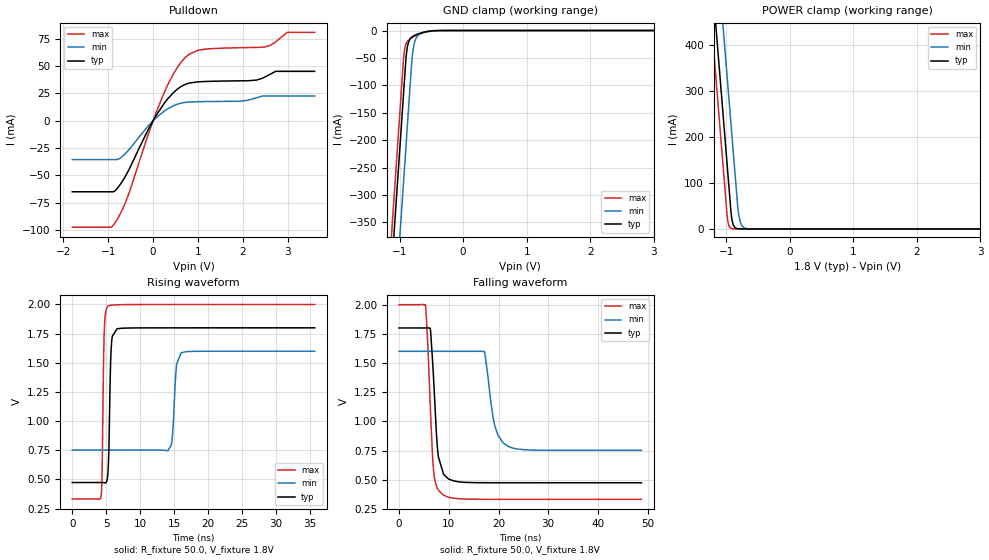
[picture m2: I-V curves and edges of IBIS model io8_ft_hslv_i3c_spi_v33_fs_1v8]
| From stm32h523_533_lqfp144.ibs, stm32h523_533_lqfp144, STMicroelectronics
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[Model]   io8_ft_hslv_i3c_spi_v33_fs_1v8
Model_type I/O_open_drain
Polarity   Non-Inverting
Enable   Active-Low
| CAP_THRESHOLD on pad IOFT is "UDTCAPC" :
| Rising=20.0% of vddiom   Falling=80.0% of vddiom
| C_comp min and max val. don't necessarily correlate with the min and max pvt
| but are the smallest and greatest pad capacitance found.
| var   typ   min   max
C_comp   3.69213pF  3.66975pF  3.86731pF
|C_comp_pulldown   3.69213pF  3.66975pF  3.86731pF
Vinl = 800.0mV
Vinh = 1.0V
Vmeas = 900.0mV   | Reference voltage for timing measurements
Cref  = 50.0pF   | Timing specification test load capacitance value
Rref  = 1.0MOhm   | Timing specification test load resistance value
Vref  = 990.0mV   | Timing specification test load voltage
[Model Spec]
| TIME_THRESHOLD on pin ZII2CV11 is "CMOS" :
| Rising=40.0% of vdd   Falling=60.0% of vdd
Vinl 693.80000mV 621.80000mV 774.80000mV
Vinh 1.05820V 933.20000mV 1.16320V
| variable   typ   min   max
[Temperature Range] 25.0 125.0 -40.0
| variable   typ   min   max
[Voltage Range] 1.8V 1.6V 2.0V
| variable   typ   min   max
[POWER Clamp Reference] 1.8V 1.6V 2.0V
| variable   typ   min   max
[GND Clamp Reference] 0V 0V 0V
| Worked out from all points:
|   slope of the pulldown table from 0 to 0.27 V, typ, clamps not added: 15.8 ohm
|   GND clamp passes 1 mA (typ) near -0.52 V on its own axis
|   POWER clamp passes 1 mA (typ) near -0.84 V on its own axis
|   rising waveform, R_fixture 50.0, V_fixture 1.8V: 20-80 % time 287ps typ, 468ps min, 243ps max; typ from 0.474 V to 1.8 V
|   falling waveform, R_fixture 50.0, V_fixture 1.8V: 20-80 % time 1.08ns typ, 1.84ns min, 1.02ns max; typ from 1.8 V to 0.474 V
[POWER Clamp]
-1.8V     1.518A     1.709A     1.407A
-1.23V    548.8mA    740.2mA    437.5mA
-1.16V    429.8mA    621.2mA    318.5mA
-1.05V    242.8mA    434.2mA    131.5mA
-980mV    123.8mA    315.2mA    17.95mA
-930mV    38.81mA    230.2mA    1.49mA
-910mV    17.82mA    196.2mA    550.8uA
-890mV    8.18mA     162.2mA    203.5uA
-810mV    363.5uA    33.6mA     3.797uA
-770mV    76.62uA    10.47mA    518.8nA
-710mV    7.416uA    1.822mA    26.33nA
3.6V      0A         0A         0A
[GND Clamp]
-1.8V     -1.579A    -1.74A     -1.515A
-1.24V    -627.3mA   -788.3mA   -562.7mA
-1.05V    -304.3mA   -465.3mA   -239.7mA
-940mV    -117.3mA   -278.3mA   -52.69mA
-930mV    -100.3mA   -261.3mA   -40.52mA
-900mV    -50.11mA   -210.3mA   -24.23mA
-880mV    -30.95mA   -176.3mA   -20.02mA
-810mV    -12.18mA   -57.97mA   -13.23mA
-780mV    -9.807mA   -29.1mA    -11.19mA
-690mV    -5.41mA    -7.142mA   -6.184mA
-420mV    -170.4uA   -446.1uA   -81.94uA
3.6V      5.755nA    953.2nA    228.2pA
| variable   typ   min   max
[Pullup Reference] 1.8V 1.6V 2.0V
| variable   typ   min   max
[Pulldown Reference] 0V 0V 0V
[Pulldown]
-1.8V     -65.02mA   -35.56mA   -97.42mA
-940mV    -65.02mA   -35.56mA   -97.42mA
-850mV    -64.17mA   -35.56mA   -93.49mA
-570mV    -47.32mA   -28.01mA   -70.04mA
-120mV    -9.088mA   -5.279mA   -14.07mA
250mV     16.04mA    8.832mA    26.05mA
550mV     29.17mA    15.25mA    49.41mA
780mV     34.17mA    17.07mA    60.14mA
1.18V     35.97mA    17.56mA    65.65mA
2.49V     40mA       22.62mA    67.56mA
2.99V     45.21mA    22.62mA    80.94mA
3.6V      45.21mA    22.62mA    80.94mA
[Ramp]
dV/dt_r 795.76295mV/283.27367ps 508.91357mV/466.70839ps 1.00097V/238.8475ps
dV/dt_f 795.78719mV/1.07804ns 508.97957mV/1.79002ns 1.00099V/1.02285ns
R_load = 50.0
| Removed startup time: 0s 0s 0s  .
| Removed end time: 35.75ns.
[Rising Waveform]
R_fixture   = 50.0
V_fixture   = 1.8V
V_fixture_min = 1.6V
V_fixture_max = 2.0V
0s        473.7mV    751.7mV    331.7mV
4.2ns     473.8mV    751.7mV    342.5mV
4.4ns     473.6mV    751.7mV    567.3mV
4.7ns     471.9mV    751.7mV    1.739V
5.25ns    548.8mV    751.7mV    1.984V
5.75ns    1.634V     751.7mV    1.994V
6.6ns     1.792V     751.7mV    1.997V
14.1ns    1.8V       746.3mV    2V
16.05ns   1.8V       1.587V     2V
35.75ns   1.8V       1.6V       2V
| Removed startup time: 0s 0s 0s  .
| Removed end time: 48.75ns.
[Falling Waveform]
R_fixture   = 50.0
V_fixture   = 1.8V
V_fixture_min = 1.6V
V_fixture_max = 2.0V
0s        1.8V       1.6V       2V
5.3ns     1.8V       1.6V       1.998V
6.3ns     1.787V     1.6V       1.104V
6.95ns    1.357V     1.6V       569.4mV
7.8ns     732.9mV    1.6V       417.7mV
8.95ns    545.1mV    1.6V       366.6mV
17.15ns   474mV      1.597V     332mV
19.25ns   473.8mV    961.4mV    331.8mV
21.9ns    473.7mV    785.9mV    331.7mV
48.75ns   473.7mV    751.7mV    331.7mV
